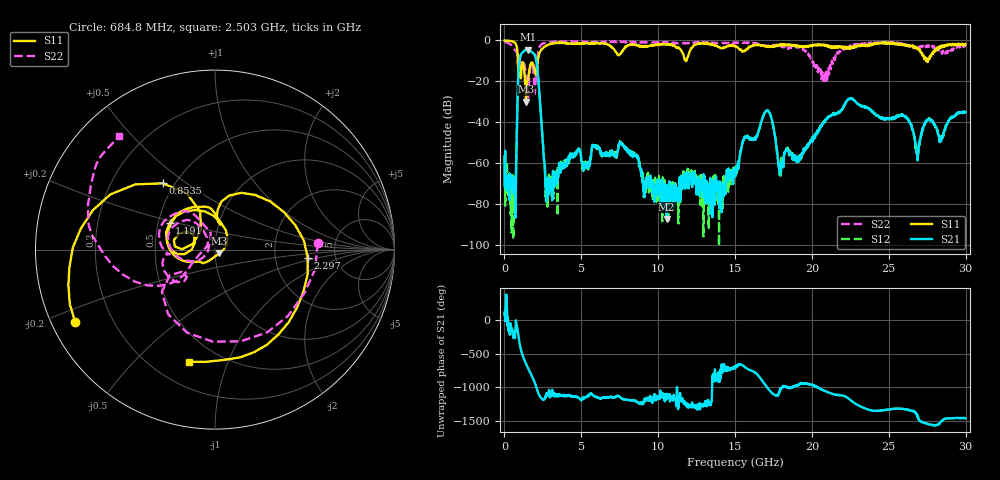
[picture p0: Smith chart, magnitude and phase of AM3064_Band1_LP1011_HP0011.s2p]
# Hz S DB R 50.0
!freq dBS11 angS11 dBS21 angS21 dBS12 angS12 dBS22 angS22
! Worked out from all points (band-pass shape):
!   1600 points, 10 MHz to 29.98 GHz, reference 50 ohm
!   highest |S21| = -4.45 dB at 1.51 GHz (marker M1); lowest = -87.3 dB at 10.54 GHz (marker M2)
!   |S21| within 3 dB of the highest: 1.044 GHz to 1.986 GHz (941.8 MHz wide, 62.2 % of centre)
!   lowest |S11| = -29.9 dB at 1.397 GHz (marker M3), VSWR 1.07, Z = 52.5 - j2.16 ohm
!   |S11| at or under -10 dB: 876.6 MHz to 2.168 GHz (1.292 GHz wide, 84.8 % of centre); 11.79413 GHz to 11.83906 GHz (44.93 MHz wide, 0.38 % of centre); 27.41247 GHz to 27.43594 GHz (23.47 MHz wide, 0.0856 % of centre)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
!   |S22| runs from -28.7 to -0.3 dB; largest |S21 - S12| = 0.0082
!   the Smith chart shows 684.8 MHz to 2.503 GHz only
!   S11 on the Smith chart (normalised r, x): 684.8 MHz: 0.07, -0.24; 853.5 MHz: 0.43, +0.41; 1.191 GHz: 0.57, +0.18; 2.297 GHz: 3.10, -0.37; 2.503 GHz: 0.35, -0.73
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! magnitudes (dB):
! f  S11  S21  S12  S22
! 10 MHz  0.0  -56.7  -56.1  -0.3
! 684.8 MHz  -1.1  -73.4  -71.4  -4.8
! 853.5 MHz  -6.6  -27.9  -27.9  -8.4
! 984.7 MHz  -12.6  -9.4  -9.4  -10.3
! 1.191 GHz  -10.7  -5.8  -5.7  -9.6
! 1.397 GHz  -29.9  -4.5  -4.5  -17.3
! 1.51 GHz  -19.5  -4.5  -4.4  -25.8
! 2.297 GHz  -5.7  -28.6  -28.5  -2.9
! 2.503 GHz  -3.9  -50.7  -50.5  -1.7
! 2.822 GHz  -2.2  -69.4  -79.2  -1.0
! 5.015 GHz  -1.5  -59.1  -59.1  -0.7
! 7.601 GHz  -6.1  -50.2  -49.4  -0.7
! 10 GHz  -2.0  -71.2  -72.0  -1.0
! 10.54 GHz  -2.2  -87.3  -75.9  -1.2
! 15 GHz  -2.8  -66.0  -64.1  -1.4
! 17.05 GHz  -2.8  -34.3  -34.0  -2.8
! 17.97 GHz  -2.4  -62.9  -66.2  -2.7
! 19.99 GHz  -2.8  -48.6  -49.1  -9.4
! 22.45 GHz  -3.1  -28.6  -28.4  -3.5
! 25 GHz  -1.1  -38.3  -38.5  -1.1
! 26.87 GHz  -4.1  -58.7  -57.6  -3.1
! 29.98 GHz  -1.9  -35.1  -34.8  -3.1
